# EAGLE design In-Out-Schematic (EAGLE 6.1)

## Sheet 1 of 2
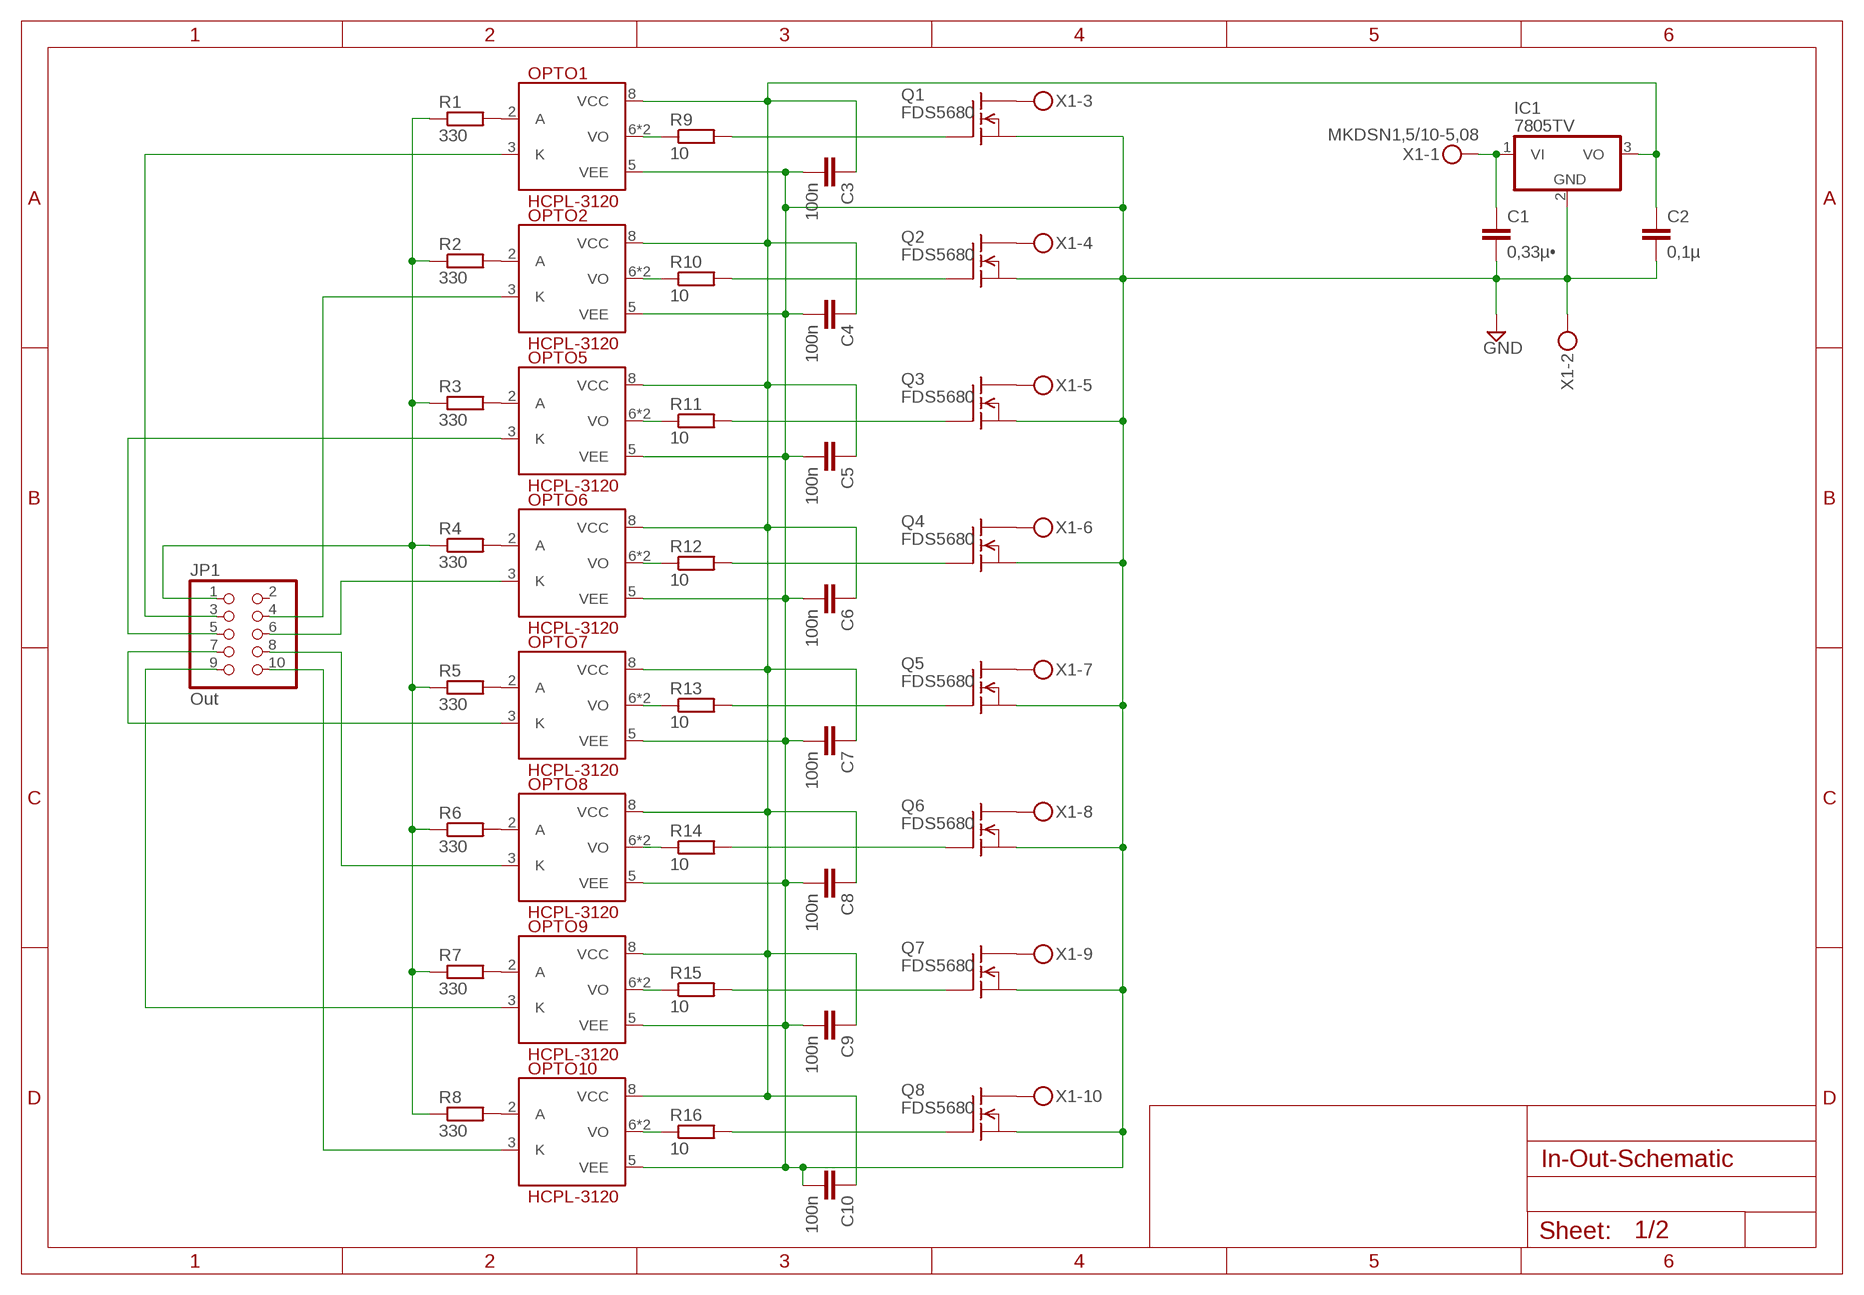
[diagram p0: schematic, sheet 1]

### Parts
C1  0,33µ•  C-EUC0805  [C0805]
C2  0,1µ  C-EUC0402  [C0402]
C3  100n  C-EUC0402  [C0402]
C4  100n  C-EUC0402  [C0402]
C5  100n  C-EUC0402  [C0402]
C6  100n  C-EUC0402  [C0402]
C7  100n  C-EUC0402  [C0402]
C8  100n  C-EUC0402  [C0402]
C9  100n  C-EUC0402  [C0402]
C10  100n  C-EUC0402  [C0402]
IC1  7805TV  [TO220V]
JP1  Out  PINHD-2X5  [2X05]
OPTO1  HCPL-3120  [HCPL-3120-SOIC-8]
OPTO2  HCPL-3120  [HCPL-3120-SOIC-8]
OPTO5  HCPL-3120  [HCPL-3120-SOIC-8]
OPTO6  HCPL-3120  [HCPL-3120-SOIC-8]
OPTO7  HCPL-3120  [HCPL-3120-SOIC-8]
OPTO8  HCPL-3120  [HCPL-3120-SOIC-8]
OPTO9  HCPL-3120  [HCPL-3120-SOIC-8]
OPTO10  HCPL-3120  [HCPL-3120-SOIC-8]
Q1  FDS5680  [SO-8]
Q2  FDS5680  [SO-8]
Q3  FDS5680  [SO-8]
Q4  FDS5680  [SO-8]
Q5  FDS5680  [SO-8]
Q6  FDS5680  [SO-8]
Q7  FDS5680  [SO-8]
Q8  FDS5680  [SO-8]
R1  330  R-EU_R0603  [R0603]
R2  330  R-EU_R0603  [R0603]
R3  330  R-EU_R0603  [R0603]
R4  330  R-EU_R0603  [R0603]
R5  330  R-EU_R0603  [R0603]
R6  330  R-EU_R0603  [R0603]
R7  330  R-EU_R0603  [R0603]
R8  330  R-EU_R0603  [R0603]
R9  10  R-EU_R1206  [R1206]
R10  10  R-EU_R1206  [R1206]
R11  10  R-EU_R1206  [R1206]
R12  10  R-EU_R1206  [R1206]
R13  10  R-EU_R1206  [R1206]
R14  10  R-EU_R1206  [R1206]
R15  10  R-EU_R1206  [R1206]
R16  10  R-EU_R1206  [R1206]
X1  MKDSN1,5/10-5,08  [MKDSN1,5/10-5,08]

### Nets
GND: C1.2 C2.2 C3.2 C4.2 C5.2 C6.2 C7.2 C8.2 C9.2 C10.2 IC1.2(GND) OPTO1.5(VEE) OPTO2.5(VEE) OPTO5.5(VEE) OPTO6.5(VEE) OPTO7.5(VEE) OPTO8.5(VEE) OPTO9.5(VEE) OPTO10.5(VEE) Q1.1(S) Q1.2(S) Q1.3(S) Q2.1(S) Q2.2(S) Q2.3(S) Q3.1(S) Q3.2(S) Q3.3(S) Q4.1(S) Q4.2(S) Q4.3(S) Q5.1(S) Q5.2(S) Q5.3(S) Q6.1(S) Q6.2(S) Q6.3(S) Q7.1(S) Q7.2(S) Q7.3(S) Q8.1(S) Q8.2(S) Q8.3(S) X1.2
N$2 [Power]: C1.1 IC1.1(VI) X1.1
N$3: Q1.5(D) Q1.6(D) Q1.7(D) Q1.8(D) X1.3
N$4: Q2.5(D) Q2.6(D) Q2.7(D) Q2.8(D) X1.4
N$5: Q3.5(D) Q3.6(D) Q3.7(D) Q3.8(D) X1.5
N$6: Q4.5(D) Q4.6(D) Q4.7(D) Q4.8(D) X1.6
N$7: Q5.5(D) Q5.6(D) Q5.7(D) Q5.8(D) X1.7
N$8: Q6.5(D) Q6.6(D) Q6.7(D) Q6.8(D) X1.8
N$9: Q7.5(D) Q7.6(D) Q7.7(D) Q7.8(D) X1.9
N$10: Q8.5(D) Q8.6(D) Q8.7(D) Q8.8(D) X1.10
N$11: OPTO1.2(A) R1.2
N$12: OPTO2.2(A) R2.2
N$13: OPTO5.2(A) R3.2
N$14: OPTO6.2(A) R4.2
N$15: OPTO7.2(A) R5.2
N$16: OPTO8.2(A) R6.2
N$17: OPTO9.2(A) R7.2
N$18: OPTO10.2(A) R8.2
N$19: JP1.1 R1.1 R2.1 R3.1 R4.1 R5.1 R6.1 R7.1 R8.1
N$20: JP1.5 OPTO5.3(K)
N$21: JP1.3 OPTO1.3(K)
N$22: JP1.4 OPTO2.3(K)
N$23: JP1.6 OPTO6.3(K)
N$24: JP1.7 OPTO7.3(K)
N$25: JP1.8 OPTO8.3(K)
N$26: JP1.9 OPTO9.3(K)
N$27: JP1.10 OPTO10.3(K)
N$28: OPTO1.6(VO) OPTO1.7(VO) R9.1
N$29: Q1.4(G) R9.2
N$30: OPTO2.6(VO) OPTO2.7(VO) R10.1
N$31: Q2.4(G) R10.2
N$32: OPTO5.6(VO) OPTO5.7(VO) R11.1
N$33: Q3.4(G) R11.2
N$34: OPTO6.6(VO) OPTO6.7(VO) R12.1
N$35: Q4.4(G) R12.2
N$36: OPTO7.6(VO) OPTO7.7(VO) R13.1
N$37: Q5.4(G) R13.2
N$38: Q6.4(G) R14.2
N$39: OPTO8.6(VO) OPTO8.7(VO) R14.1
N$40: OPTO9.6(VO) OPTO9.7(VO) R15.1
N$41: Q7.4(G) R15.2
N$42: OPTO10.6(VO) OPTO10.7(VO) R16.1
N$59: Q8.4(G) R16.2
N$71 [Power]: C2.1 C3.1 C4.1 C5.1 C6.1 C7.1 C8.1 C9.1 C10.1 IC1.3(VO) OPTO1.8(VCC) OPTO2.8(VCC) OPTO5.8(VCC) OPTO6.8(VCC) OPTO7.8(VCC) OPTO8.8(VCC) OPTO9.8(VCC) OPTO10.8(VCC)
Unconnected: JP1.2

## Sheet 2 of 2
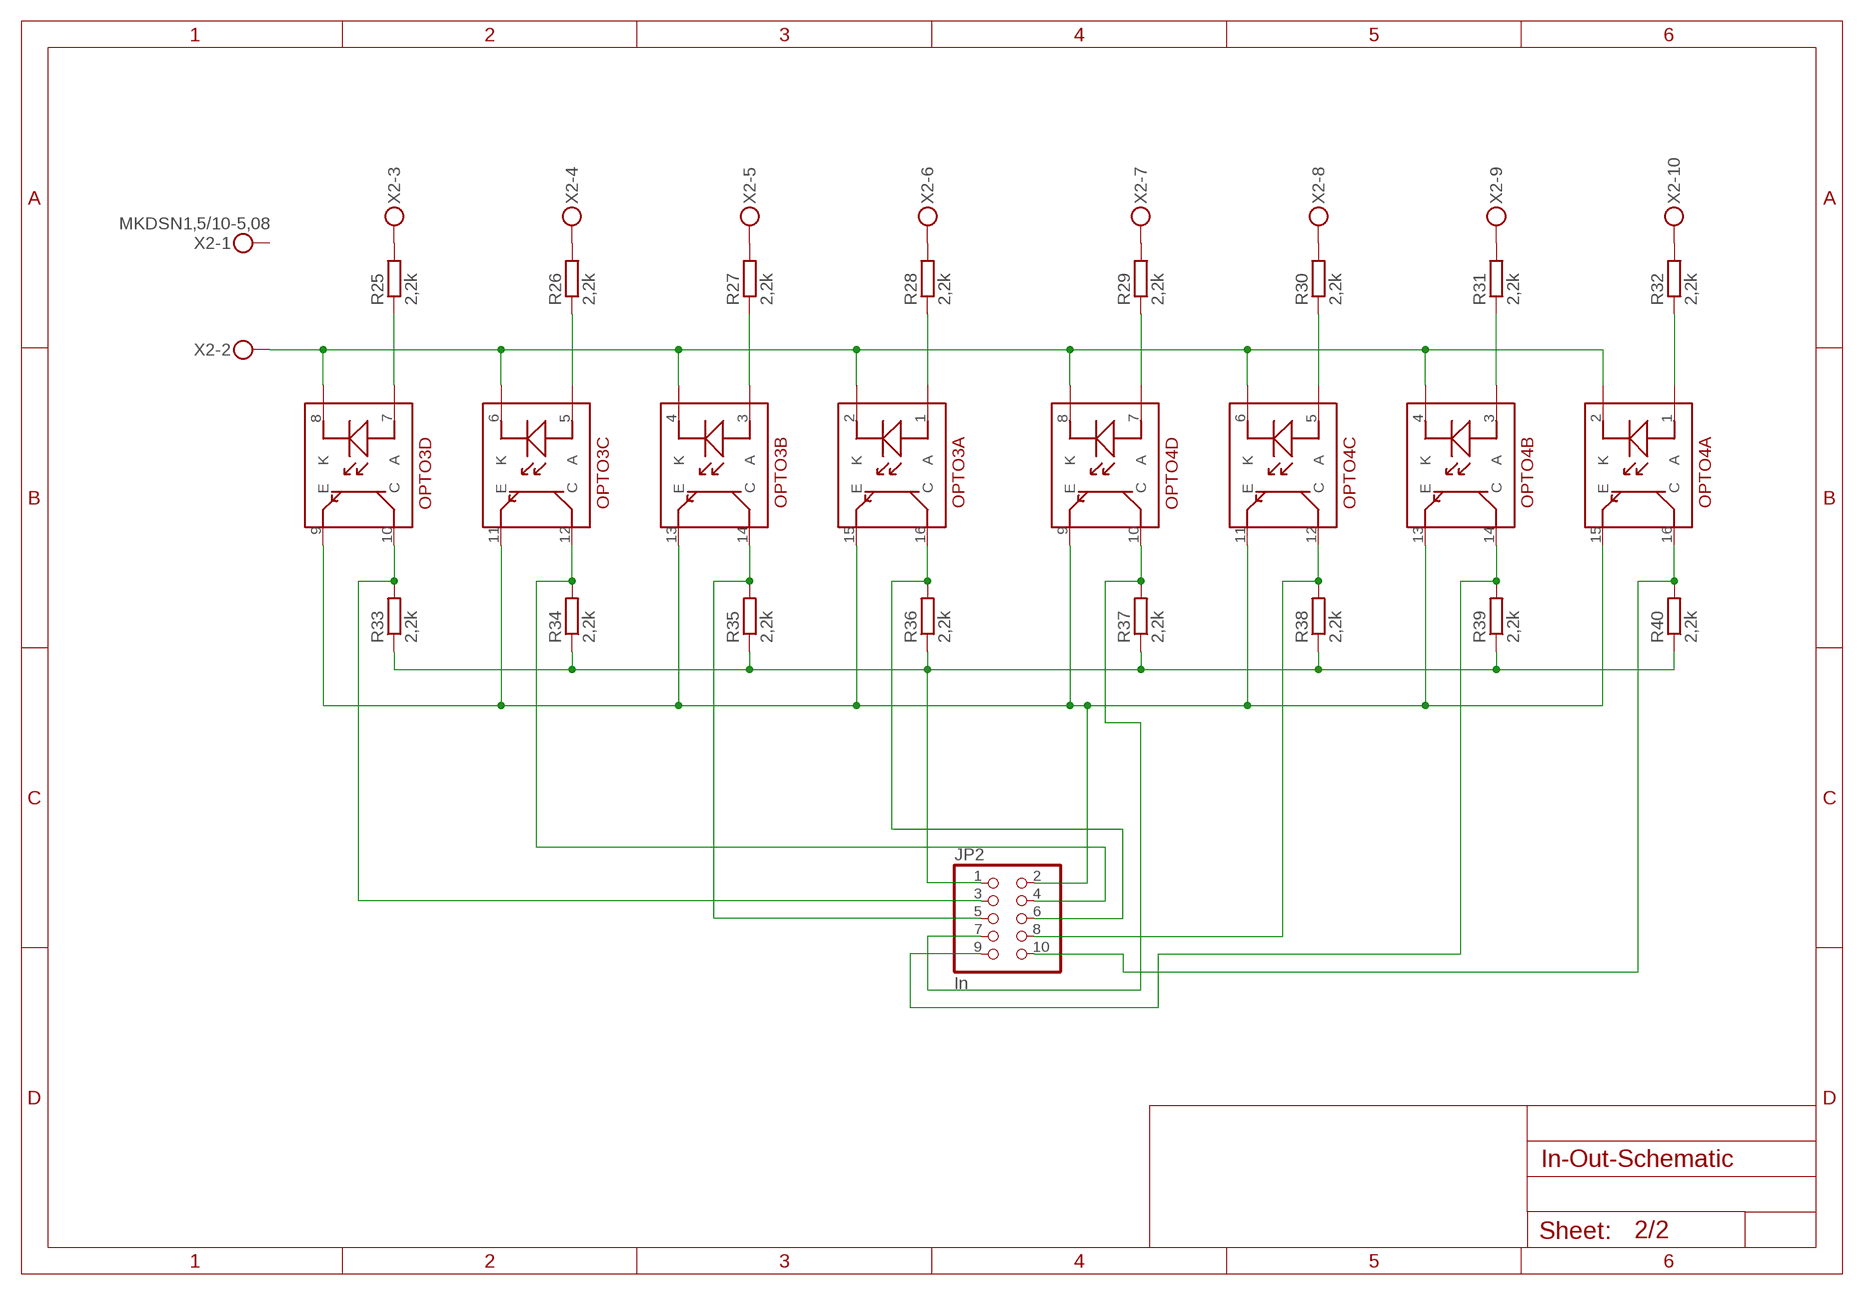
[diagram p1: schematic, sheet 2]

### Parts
JP2  In  PINHD-2X5  [2X05]
OPTO3  QUAD-OPTO_ACPL-247  [SOIC-16]
OPTO4  QUAD-OPTO_ACPL-247  [SOIC-16]
R25  2,2k  R-EU_R0805  [R0805]
R26  2,2k  R-EU_R0805  [R0805]
R27  2,2k  R-EU_R0805  [R0805]
R28  2,2k  R-EU_R0805  [R0805]
R29  2,2k  R-EU_R0805  [R0805]
R30  2,2k  R-EU_R0805  [R0805]
R31  2,2k  R-EU_R0805  [R0805]
R32  2,2k  R-EU_R0805  [R0805]
R33  2,2k  R-EU_R0805  [R0805]
R34  2,2k  R-EU_R0805  [R0805]
R35  2,2k  R-EU_R0805  [R0805]
R36  2,2k  R-EU_R0805  [R0805]
R37  2,2k  R-EU_R0805  [R0805]
R38  2,2k  R-EU_R0805  [R0805]
R39  2,2k  R-EU_R0805  [R0805]
R40  2,2k  R-EU_R0805  [R0805]
X2  MKDSN1,5/10-5,08  [MKDSN1,5/10-5,08]

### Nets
N$43: OPTO3.7(D:A) R25.1
N$44: OPTO3.1(A:A) R28.1
N$45: OPTO3.5(C:A) R26.1
N$46: OPTO3.3(B:A) R27.1
N$47: OPTO3.2(A:K) OPTO3.4(B:K) OPTO3.6(C:K) OPTO3.8(D:K) OPTO4.2(A:K) OPTO4.4(B:K) OPTO4.6(C:K) OPTO4.8(D:K) X2.2
N$48: OPTO4.7(D:A) R29.1
N$49: OPTO4.5(C:A) R30.1
N$50: OPTO4.3(B:A) R31.1
N$51: OPTO4.1(A:A) R32.1
N$52: JP2.3 OPTO3.10(D:C) R33.2
N$53: JP2.4 OPTO3.12(C:C) R34.2
N$54: JP2.5 OPTO3.14(B:C) R35.2
N$55: JP2.6 OPTO3.16(A:C) R36.2
N$56: JP2.7 OPTO4.10(D:C) R37.2
N$57: JP2.8 OPTO4.12(C:C) R38.2
N$58: JP2.10 OPTO4.16(A:C) R40.2
N$60: R25.2 X2.3
N$61: R26.2 X2.4
N$62: R27.2 X2.5
N$63: R28.2 X2.6
N$64: R29.2 X2.7
N$65: R30.2 X2.8
N$66: R31.2 X2.9
N$67: R32.2 X2.10
N$68: JP2.1 R33.1 R34.1 R35.1 R36.1 R37.1 R38.1 R39.1 R40.1
N$69: JP2.2 OPTO3.9(D:E) OPTO3.11(C:E) OPTO3.13(B:E) OPTO3.15(A:E) OPTO4.9(D:E) OPTO4.11(C:E) OPTO4.13(B:E) OPTO4.15(A:E)
N$77: JP2.9 OPTO4.14(B:C) R39.2
Unconnected: X2.1

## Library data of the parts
C1-C10 = rcl:C-EU: CAPACITOR, European symbol
IC1 = linear:78*: Positive VOLTAGE REGULATOR Source: http://cache.national.com/ds/LM/LM78L05.pdf http://www.fairchildsemi.com/ds/LM/LM7805.pdf
JP1 JP2 = pinhead:PINHD-2X5: PIN HEADER
OPTO1 OPTO2 OPTO5-OPTO10 = Bachelorarbeit_lib_Jonas:HCPL-3120: HCPL-3120 Gate Driver Opto
OPTO3 OPTO4 = Bachelorarbeit_lib_Jonas:QUAD-OPTO_ACPL-247: 4-fach Optokoppler AVAGO ACPL-247 SOIC-16 Package
Q1-Q8 = transistor-fet:FDS5680: 60V N-Channel PowerTrench TM MOSFET FAIRCHILD FDS5680.pdf
R1-R16 R25-R40 = rcl:R-EU_: RESISTOR, European symbol
X1 X2 = con-phoenix-508:MKDSN1,5/10-5,08: MKDSN 1,5/10-5,08 Printklemme Nennstrom: 13,5 A Nennspannung: 250 V Rastermaß: 5,08 mm Polzahl: 10 Anschlussart: Schraubanschluss Montage: Löten Anschlussrichtung Leiter/Platine: 0 ° Artikelnummer: 1729209 Source: http://eshop.phoenixcontact.com .. 1729209.pdf; MPN: SMKDSN1,5/10-5,08; OC_FARNELL: 1792913; OC_NEWARK: 70R0297

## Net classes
1 Power: width 0.508 mm, clearance 0.305 mm

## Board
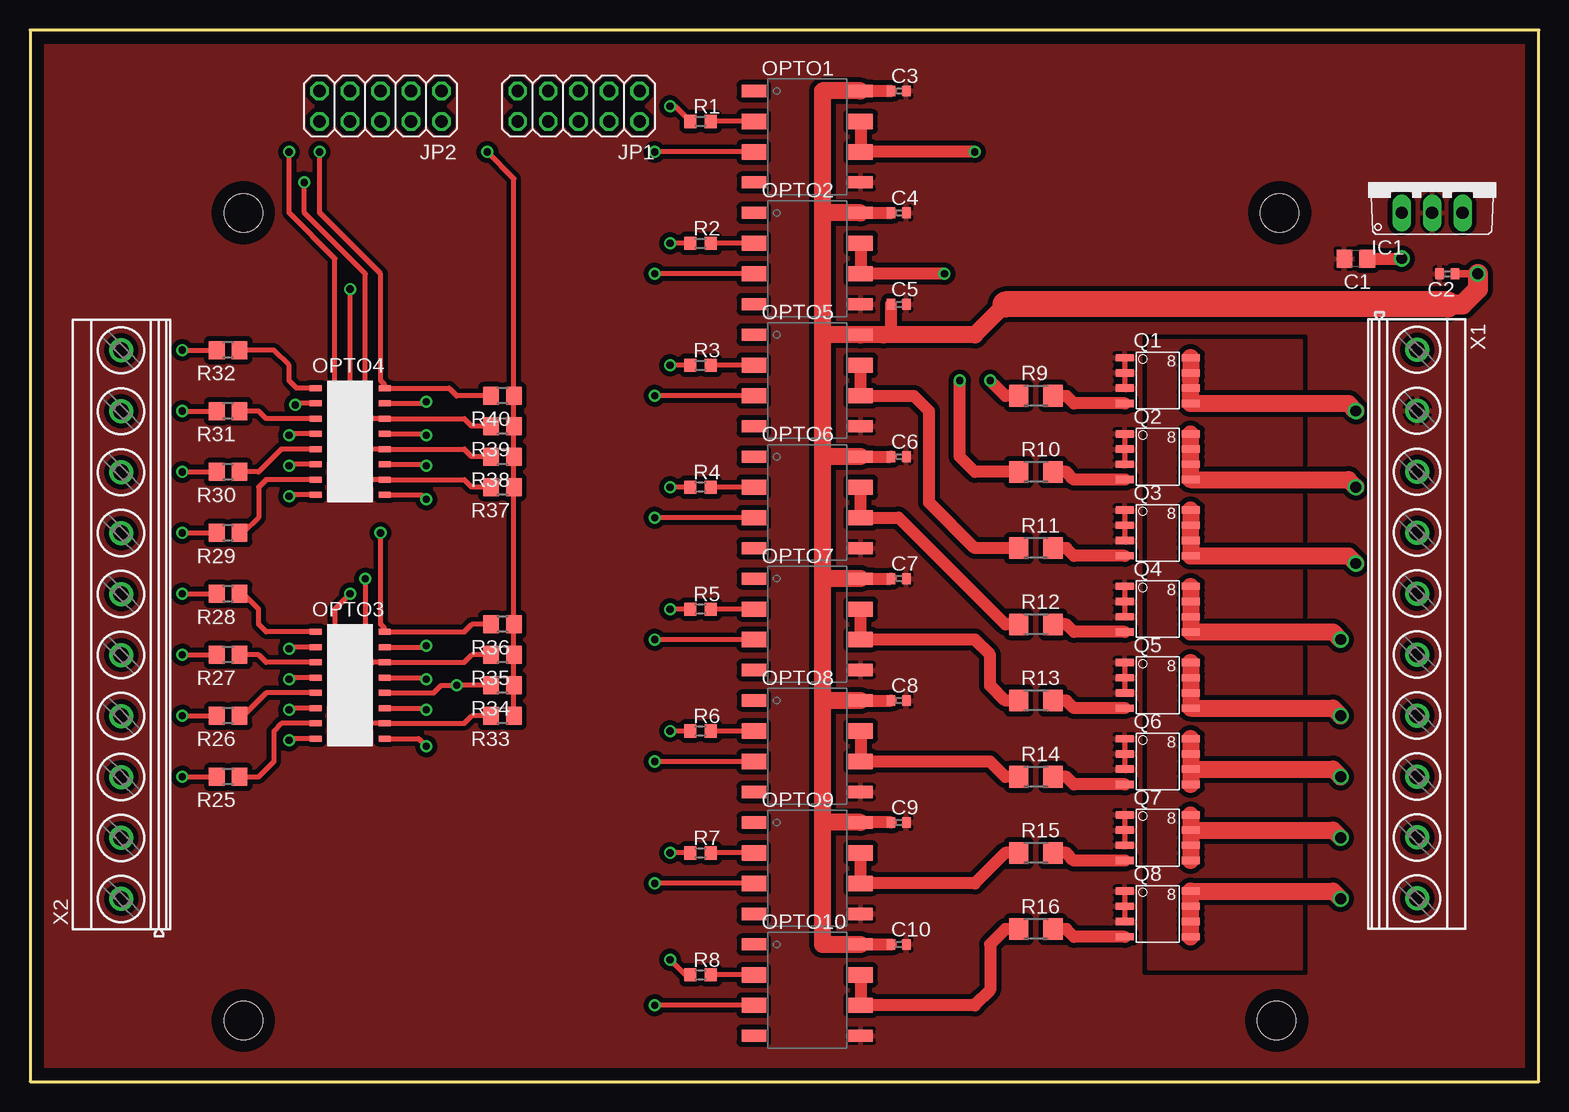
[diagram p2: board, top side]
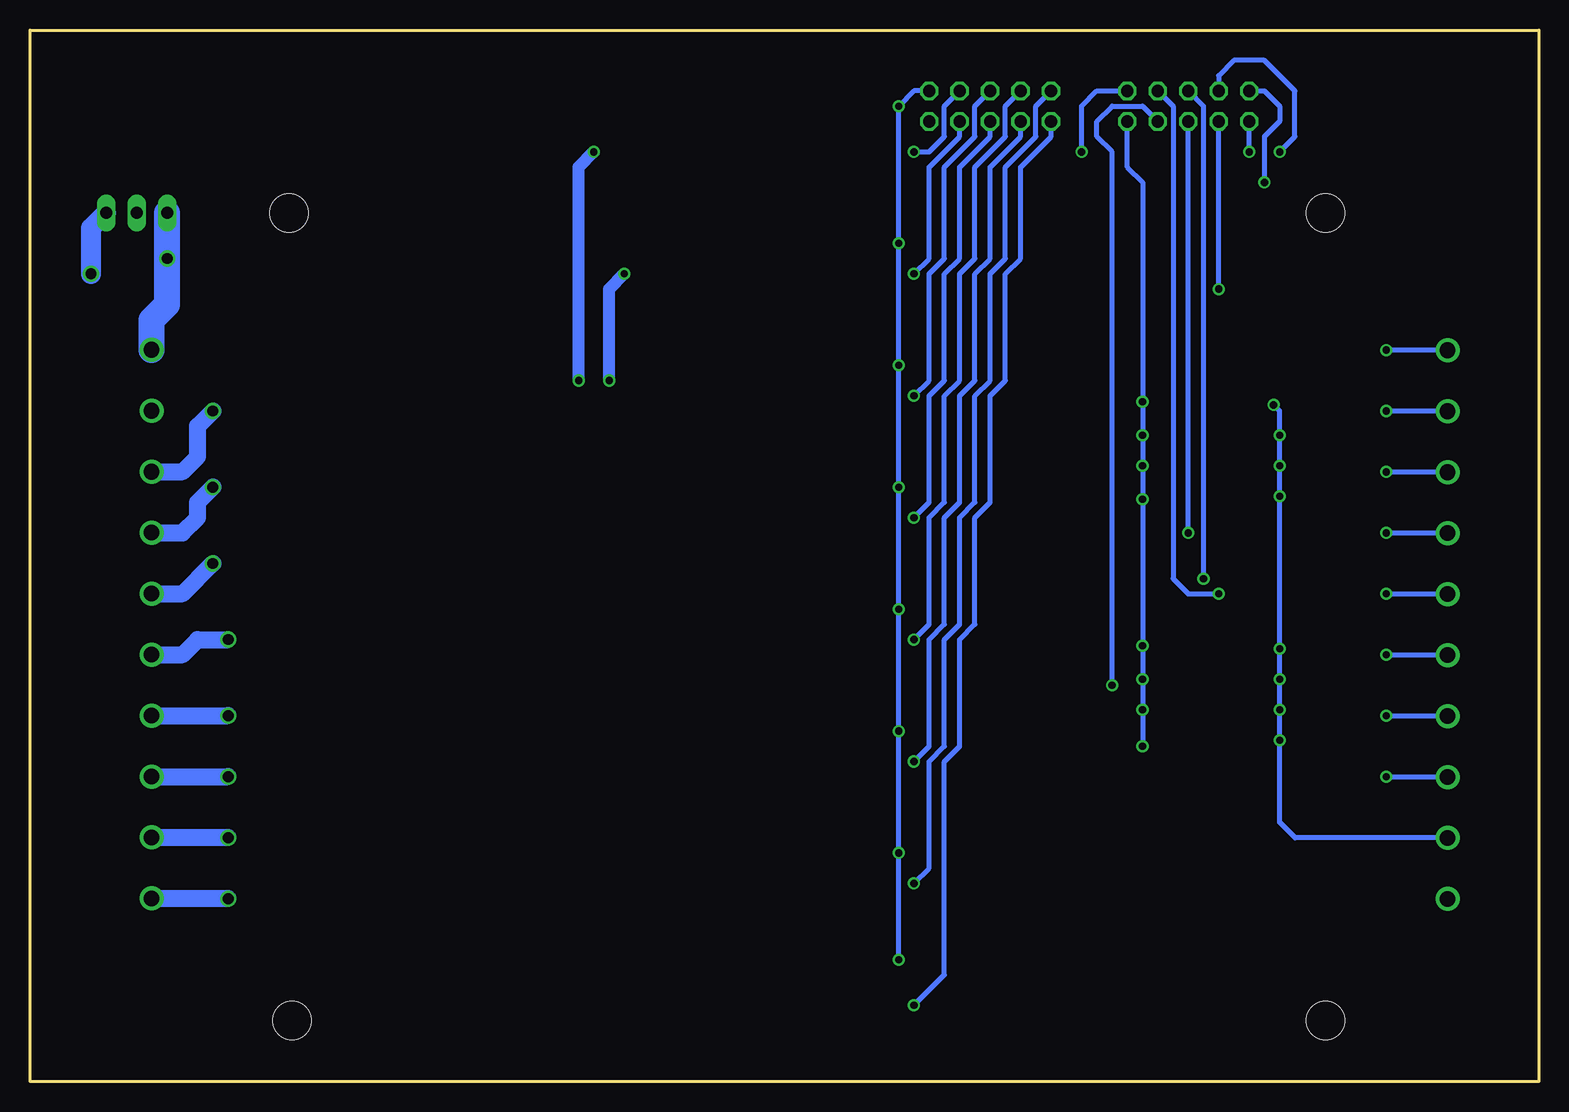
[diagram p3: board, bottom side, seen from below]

Size 125.73 x 87.63 mm. Coordinates in mm from the lower left corner, seen from the top.
Outline: 0,0 125.73,0 125.73,87.63 0,87.63 0,0
Copper layers (1*16): Top 0.035mm / dielectric 1.5mm / Bottom 0.035mm
Design rules: minimum track width 10mil, minimum drill 23mil, track to track 16mil, track to pad 12mil, pad to pad 16mil, via to via 16mil, smd to smd 8mil, copper to edge 40mil, drill to drill 8mil, minimum pad ring 10mil, minimum via ring 8mil, stop-mask expansion 4mil, vias tented up to drill 0mil, thermal gap 10mil
Holes 3.2 mm at 17.78,5.08 17.78,72.39 103.89,5.08 104.14,72.39

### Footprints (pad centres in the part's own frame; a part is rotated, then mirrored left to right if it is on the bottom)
C0805 = smd 1.3 x 1.5: 1 -0.95,0; 2 0.95,0
C0402 = smd 0.7 x 0.9: 1 -0.65,0; 2 0.65,0
TO220V = drill 1.016 long: 1 -2.54,-2.54; 2 0,-2.54; 3 2.54,-2.54
2X05 = drill 1.016 octagon: 1 -5.08,-1.27; 2 -5.08,1.27; 3 -2.54,-1.27; 4 -2.54,1.27; 5 0,-1.27; 6 0,1.27; 7 2.54,-1.27; 8 2.54,1.27; 9 5.08,-1.27; 10 5.08,1.27
HCPL-3120-SOIC-8 = smd 1.016 x 2.032: 1 -3.81,-4.445; 4 3.81,-4.445; 5 3.81,4.445; 8 -3.81,4.445 | smd 1.27 x 2.032: 2 -1.27,-4.445; 3 1.27,-4.445; 6 1.27,4.445; 7 -1.27,4.445
SOIC-16 = smd 0.5 x 1: 1 -4.445,-2.875; 2 -3.175,-2.875; 3 -1.905,-2.875; 4 -0.635,-2.875; 5 0.635,-2.875; 6 1.905,-2.875; 7 3.175,-2.875; 8 4.445,-2.875; 9 4.445,2.875; 10 3.175,2.875; 11 1.905,2.875; 12 0.635,2.875; 13 -0.635,2.875; 14 -1.905,2.875; 15 -3.175,2.875; 16 -4.445,2.875
SO-8 = smd 1.524 x 0.61: 1 -2.743,1.905; 2 -2.743,0.635; 3 -2.743,-0.635; 4 -2.743,-1.905; 5 2.743,-1.905; 6 2.743,-0.635; 7 2.743,0.635; 8 2.743,1.905
R0603 = smd 1 x 1.1: 1 -0.85,0; 2 0.85,0
R1206 = smd 1.6 x 1.803: 1 -1.422,0; 2 1.422,0
R0805 = smd 1.3 x 1.5: 1 -0.95,0; 2 0.95,0
MKDSN1,5/10-5,08 = drill 1.3 pad 2: 1 -22.881,0.025; 2 -17.801,0.025; 3 -12.721,0.025; 4 -7.641,0.025; 5 -2.561,0.025; 6 2.519,0.025; 7 7.599,0.025; 8 12.679,0.025; 9 17.759,0.025; 10 22.839,0.025

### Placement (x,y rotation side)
C1  110.49,68.58 180 top
C2  118.11,67.31 180 top
C3  72.39,82.55 0 top
C4  72.39,72.39 0 top
C5  72.39,64.77 0 top
C6  72.39,52.07 0 top
C7  72.39,41.91 0 top
C8  72.39,31.75 0 top
C9  72.39,21.59 0 top
C10  72.39,11.43 0 top
IC1  116.84,74.93 0 top
JP1  45.72,81.28 180 top
JP2  29.21,81.28 180 top
OPTO1  64.77,78.74 270 top
OPTO2  64.77,68.58 270 top
OPTO3  26.67,33.02 270 top
OPTO4  26.67,53.34 270 top
OPTO5  64.77,58.42 270 top
OPTO6  64.77,48.26 270 top
OPTO7  64.77,38.1 270 top
OPTO8  64.77,27.94 270 top
OPTO9  64.77,17.78 270 top
OPTO10  64.77,7.62 270 top
Q1  93.98,58.42 0 top
Q2  93.98,52.07 0 top
Q3  93.98,45.72 0 top
Q4  93.98,39.37 0 top
Q5  93.98,33.02 0 top
Q6  93.98,26.67 0 top
Q7  93.98,20.32 0 top
Q8  93.98,13.97 0 top
R1  55.88,80.01 0 top
R2  55.88,69.85 0 top
R3  55.88,59.69 0 top
R4  55.88,49.53 0 top
R5  55.88,39.37 0 top
R6  55.88,29.21 0 top
R7  55.88,19.05 0 top
R8  55.88,8.89 0 top
R9  83.82,57.15 0 top
R10  83.82,50.8 0 top
R11  83.82,44.45 0 top
R12  83.82,38.1 0 top
R13  83.82,31.75 0 top
R14  83.82,25.4 0 top
R15  83.82,19.05 0 top
R16  83.82,12.7 0 top
R25  16.51,25.4 180 top
R26  16.51,30.48 180 top
R27  16.51,35.56 180 top
R28  16.51,40.64 180 top
R29  16.51,45.72 180 top
R30  16.51,50.8 180 top
R31  16.51,55.88 180 top
R32  16.51,60.96 180 top
R33  39.37,30.48 180 top
R34  39.37,33.02 180 top
R35  39.37,35.56 180 top
R36  39.37,38.1 180 top
R37  39.37,49.53 180 top
R38  39.37,52.07 180 top
R39  39.37,54.61 180 top
R40  39.37,57.15 180 top
X1  115.57,38.1 270 top
X2  7.62,38.1 90 top

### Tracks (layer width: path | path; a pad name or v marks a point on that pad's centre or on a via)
COOLAREA
  pour Top (rank 2, no thermals): 93.47,61.72 105.92,61.72 105.92,53.85 105.92,41.15 105.92,28.7 105.92,17.27 105.92,9.4 93.47,9.4 93.22,9.4 93.22,16.76 93.22,25.91 93.22,38.86 93.22,51.56 93.22,61.72
GND
  Top 0.406: Q1.1 Q1.2 Q1.3 | Q2.1 Q2.2 Q2.3 | Q3.1 Q3.2 Q3.3 | Q4.1 Q4.2 Q4.3 | Q5.1 Q5.2 Q5.3 | Q6.1 Q6.2 Q6.3 | Q7.1 Q7.2 Q7.3 | Q8.1 Q8.2 Q8.3
  pour Top (rank 6): 1.27,1.27 124.46,1.27 124.46,86.36 1.27,86.36
N$2  (via drill 0.9)
  Top 1.016: C1.1 v114.3,68.58
  Bottom 2.184: X1.1 115.59,63.48 114.3,64.77 v114.3,68.58 IC1.1
N$3  (via drill 0.9)
  Top 0.406: Q1.6 96.72,58.42
  Top 1.422: v110.49,55.88 109.85,56.52 Q1.5 Q1.6 | 96.72,58.42 Q1.7 Q1.8
  Bottom 1.422: X1.3 113.01,50.82 111.76,52.07 111.76,54.61 v110.49,55.88
N$4  (via drill 0.9)
  Top 1.422: v110.49,49.53 109.85,50.17 Q2.5 Q2.6 Q2.7 Q2.8
  Bottom 0.406: 113.05,45.74 113.03,45.72
  Bottom 1.422: X1.4 113.05,45.74 | 113.03,45.72 111.76,46.99 111.76,48.26 v110.49,49.53
N$5  (via drill 0.9)
  Top 1.422: Q3.8 Q3.7 Q3.6 Q3.5 109.85,43.82 v110.49,43.18
  Bottom 1.422: X1.5 113.01,40.66 v110.49,43.18
N$6  (via drill 0.9)
  Top 1.422: Q4.8 Q4.7 Q4.6 Q4.5 108.58,37.47 v109.22,36.83
  Bottom 1.422: X1.6 113.01,35.58 111.76,36.83 v109.22,36.83
N$7  (via drill 0.9)
  Top 1.422: Q5.8 Q5.7 Q5.6 Q5.5 108.58,31.11 v109.22,30.48
  Bottom 0.406: 109.24,30.5 v109.22,30.48
  Bottom 1.422: X1.7 109.24,30.5
N$8  (via drill 0.9)
  Top 1.422: Q6.8 Q6.7 Q6.6 | Q6.6 Q6.5 | Q6.6 108.58,26.04 v109.22,25.4
  Bottom 0.406: 109.24,25.42 v109.22,25.4
  Bottom 1.422: X1.8 109.24,25.42
N$9  (via drill 0.9)
  Top 1.422: Q7.8 Q7.7 | Q7.7 Q7.6 Q7.5 | Q7.7 108.58,20.95 v109.22,20.32
  Bottom 0.406: 109.24,20.34 v109.22,20.32
  Bottom 1.422: X1.9 109.24,20.34
N$10  (via drill 0.9)
  Top 1.422: Q8.5 Q8.6 Q8.7 Q8.8 108.58,15.88 v109.22,15.24
  Bottom 0.406: 109.24,15.26 v109.22,15.24
  Bottom 1.422: X1.10 109.24,15.26
N$11
  Top 0.406: OPTO1.2 R1.2
N$12
  Top 0.406: OPTO2.2 R2.2
N$13
  Top 0.406: OPTO5.2 R3.2
N$14
  Top 0.406: OPTO6.2 R4.2
N$15
  Top 0.406: OPTO7.2 R5.2
N$16
  Top 0.406: OPTO8.2 R6.2
N$17
  Top 0.406: OPTO9.2 R7.2
N$18
  Top 0.406: OPTO10.2 R8.2
N$19  (via drill 0.6)
  Top 0.406: v53.34,81.28 53.76,81.28 R1.1 | R8.1 54.61,8.89 v53.34,10.16 | R2.1 v53.34,69.85 | R3.1 v53.34,59.69 | R4.1 v53.34,49.53 | R5.1 v53.34,39.37 | R6.1 v53.34,29.21 | R7.1 v53.34,19.05
  Bottom 0.406: JP1.1 52.07,82.55 v53.34,81.28 v53.34,69.85 v53.34,59.69 v53.34,49.53 v53.34,39.37 v53.34,29.21 v53.34,19.05 v53.34,10.16
N$20  (via drill 0.6)
  Top 0.406: OPTO5.3 v52.07,57.15
  Bottom 0.406: v52.07,57.15 50.8,58.42 50.8,67.31 49.53,68.58 49.53,76.2 46.99,78.74 46.99,81.28 JP1.5
N$21  (via drill 0.6)
  Top 0.406: OPTO1.3 v52.07,77.47
  Bottom 0.406: v52.07,77.47 50.8,77.47 49.53,78.74 49.53,81.28 JP1.3
N$22  (via drill 0.6)
  Top 0.406: OPTO2.3 v52.07,67.31
  Bottom 0.406: v52.07,67.31 50.8,68.58 50.8,76.2 48.26,78.74 JP1.4
N$23  (via drill 0.6)
  Top 0.406: OPTO6.3 v52.07,46.99
  Bottom 0.406: v52.07,46.99 50.8,48.26 50.8,57.15 49.53,58.42 49.53,67.31 48.26,68.58 48.26,76.2 45.72,78.74 JP1.6
N$24  (via drill 0.6)
  Top 0.406: OPTO7.3 v52.07,36.83
  Bottom 0.406: v52.07,36.83 50.8,38.1 50.8,46.99 49.53,48.26 49.53,57.15 48.26,58.42 48.26,67.31 46.99,68.58 46.99,76.2 44.45,78.74 44.45,81.28 JP1.7
N$25  (via drill 0.6)
  Top 0.406: OPTO8.3 v52.07,26.67
  Bottom 0.406: v52.07,26.67 50.8,27.94 50.8,36.83 49.53,38.1 49.53,46.99 48.26,48.26 48.26,57.15 46.99,58.42 46.99,67.31 45.72,68.58 45.72,76.2 43.18,78.74 JP1.8
N$26  (via drill 0.6)
  Top 0.406: OPTO9.3 v52.07,16.51
  Bottom 0.406: v52.07,16.51 50.8,17.78 50.8,26.67 49.53,27.94 49.53,36.83 48.26,38.1 48.26,46.99 46.99,48.26 46.99,57.15 45.72,58.42 45.72,67.31 44.45,68.58 44.45,76.2 41.91,78.74 41.91,81.28 JP1.9
N$27  (via drill 0.6)
  Top 0.406: OPTO10.3 v52.07,6.35
  Bottom 0.406: v52.07,6.35 49.53,8.89 49.53,26.67 48.26,27.94 48.26,36.83 46.99,38.1 46.99,46.99 45.72,48.26 45.72,57.15 44.45,58.42 44.45,67.31 43.18,68.58 43.18,76.2 40.64,78.74 JP1.10
N$28  (via drill 0.6)
  Top 1.016: R9.1 81.28,57.15 v80.01,58.42 | v78.74,77.47 OPTO1.6 OPTO1.7
  Bottom 1.016: v80.01,58.42 80.01,76.2 v78.74,77.47
N$29
  Top 1.016: R9.2 86.36,57.15 86.99,56.52 Q1.4
N$30  (via drill 0.6)
  Top 1.016: R10.1 78.74,50.8 77.47,52.07 v77.47,58.42 | v76.2,67.31 OPTO2.6 OPTO2.7
  Bottom 1.016: v77.47,58.42 77.47,66.04 v76.2,67.31
N$31
  Top 1.016: Q2.4 86.99,50.17 86.36,50.8 R10.2
N$32
  Top 1.016: R11.1 78.74,44.45 74.93,48.26 74.93,55.88 73.66,57.15 OPTO5.6 OPTO5.7
N$33
  Top 1.016: Q3.4 86.99,43.82 86.36,44.45 R11.2
N$34
  Top 1.016: OPTO6.7 OPTO6.6 72.39,46.99 81.28,38.1 R12.1
N$35
  Top 1.016: Q4.4 86.99,37.47 86.36,38.1 R12.2
N$36
  Top 1.016: R13.1 81.28,31.75 80.01,33.02 80.01,35.56 78.74,36.83 OPTO7.6 OPTO7.7
N$37
  Top 1.016: Q5.4 86.99,31.11 86.36,31.75 R13.2
N$38
  Top 1.016: Q6.4 86.99,24.77 86.36,25.4 R14.2
N$39
  Top 1.016: R14.1 81.28,25.4 80.01,26.67 OPTO8.6 OPTO8.7
N$40
  Top 1.016: R15.1 81.28,19.05 78.74,16.51 OPTO9.6 OPTO9.7
N$41
  Top 1.016: Q7.4 86.99,18.41 86.36,19.05 R15.2
N$42
  Top 1.016: R16.1 81.28,12.7 80.01,11.43 80.01,7.62 78.74,6.35 OPTO10.6 OPTO10.7
N$43
  Top 0.406: R25.1 19.05,25.4 20.32,26.67 20.32,29.21 20.95,29.84 OPTO3.7
N$44
  Top 0.406: OPTO3.1 19.68,37.47 19.05,38.1 19.05,39.37 17.78,40.64 R28.1
N$45
  Top 0.406: R26.1 17.78,30.48 19.68,32.38 OPTO3.5
N$46
  Top 0.406: OPTO3.3 19.68,34.93 19.05,35.56 R27.1
N$47  (via drill 0.6)
  Top 0.406: OPTO4.2 22.22,56.52 v22.1,56.39 | OPTO4.4 21.72,53.98 v21.59,53.85 | OPTO4.6 21.72,51.44 v21.59,51.31 | OPTO4.8 21.72,48.9 v21.59,48.77 | OPTO3.2 21.72,36.2 v21.59,36.07 | OPTO3.4 21.72,33.66 v21.59,33.53 | OPTO3.6 21.72,31.11 v21.59,30.99 | OPTO3.8 21.72,28.57 v21.59,28.45
  Bottom 0.406: X2.2 20.3,20.3 21.59,21.59 v21.59,28.45 v21.59,30.99 v21.59,33.53 v21.59,36.07 v21.59,48.77 v21.59,51.31 v21.59,53.85 21.59,55.88 v22.1,56.39
N$48
  Top 0.406: OPTO4.7 19.68,50.17 19.05,49.53 19.05,46.99 17.78,45.72 R29.1
N$49
  Top 0.406: OPTO4.5 20.95,52.71 19.05,50.8 R30.1
N$50
  Top 0.406: OPTO4.3 19.68,55.25 19.05,55.88 R31.1
N$51
  Top 0.406: OPTO4.1 22.22,57.79 21.59,58.42 21.59,59.69 20.32,60.96 R32.1
N$52  (via drill 0.6)
  Top 0.406: R33.2 36.83,30.48 36.2,29.84 OPTO3.10 27.3,29.84 25.4,31.75 25.4,39.37 v26.67,40.64
  Bottom 0.406: JP2.3 30.48,81.28 30.48,41.91 29.21,40.64 v26.67,40.64
N$53  (via drill 0.6)
  Top 0.406: OPTO3.12 33.66,32.38 34.29,33.02 v35.56,33.02 R34.2
  Bottom 0.406: v35.56,33.02 35.56,77.47 36.83,78.74 36.83,80.01 35.56,81.28 33.02,81.28 JP2.4
N$54  (via drill 0.6)
  Top 0.406: R35.2 36.83,35.56 36.2,34.93 OPTO3.14 28.57,34.93 27.94,35.56 v27.94,41.91
  Bottom 0.406: JP2.5 27.94,81.28 v27.94,41.91
N$55  (via drill 0.6)
  Top 0.406: R36.2 36.83,38.1 36.2,37.47 OPTO3.16 29.54,37.77 29.21,38.1 v29.21,45.72
  Bottom 0.406: v29.21,45.72 JP2.6
N$56  (via drill 0.6)
  Top 0.406: R37.2 36.83,49.53 36.2,50.17 OPTO4.10 27.3,50.17 25.4,52.07 25.4,68.58 21.59,72.39 v21.59,77.47
  Bottom 0.406: JP2.7 26.67,83.82 25.4,85.09 22.86,85.09 20.32,82.55 20.32,78.74 v21.59,77.47
N$57  (via drill 0.6)
  Top 0.406: R38.2 36.83,52.07 36.2,52.71 OPTO4.12 27.3,52.71 26.67,53.34 v26.67,66.04
  Bottom 0.406: v26.67,66.04 JP2.8
N$58  (via drill 0.6)
  Top 0.406: v24.13,77.47 24.13,72.39 29.21,67.31 29.21,58.42 29.54,58.09 OPTO4.16 34.93,57.79 35.56,57.15 R40.2
  Bottom 0.406: v24.13,77.47 JP2.10
N$59
  Top 1.016: Q8.4 86.99,12.06 86.36,12.7 R16.2
N$60  (via drill 0.6)
  Top 0.406: v12.7,25.4 R25.2
  Bottom 0.406: X2.3 12.68,25.38 v12.7,25.4
N$61  (via drill 0.6)
  Top 0.406: v12.7,30.48 R26.2
  Bottom 0.406: X2.4 12.68,30.46 v12.7,30.48
N$62  (via drill 0.6)
  Top 0.406: v12.7,35.56 R27.2
  Bottom 0.406: X2.5 12.68,35.54 v12.7,35.56
N$63  (via drill 0.6)
  Top 0.406: v12.7,40.64 R28.2
  Bottom 0.406: X2.6 12.68,40.62 v12.7,40.64
N$64  (via drill 0.6)
  Top 0.406: v12.7,45.72 R29.2
  Bottom 0.406: X2.7 12.68,45.7 v12.7,45.72
N$65  (via drill 0.6)
  Top 0.406: v12.7,50.8 R30.2
  Bottom 0.406: X2.8 12.68,50.78 v12.7,50.8
N$66  (via drill 0.6)
  Top 0.406: v12.7,55.88 R31.2
  Bottom 0.406: X2.9 12.68,55.86 v12.7,55.88
N$67  (via drill 0.6)
  Top 0.406: v12.7,60.96 R32.2
  Bottom 0.406: X2.10 12.68,60.94 v12.7,60.96
N$68  (via drill 0.6)
  Top 0.406: R33.1 R34.1 R35.1 R36.1 R37.1 R38.1 R39.1 R40.1 40.32,75.25 v38.1,77.47
  Bottom 0.406: v38.1,77.47 38.1,81.28 36.83,82.55 JP2.1
N$69  (via drill 0.6)
  Top 0.406: OPTO3.9 32.38,28.57 v33.02,27.94 | OPTO3.11 32.89,31.11 v33.02,30.99 | OPTO3.13 32.89,33.66 v33.02,33.53 | OPTO3.15 32.89,36.2 v33.02,36.32 | OPTO4.9 32.64,48.9 v33.02,48.51 | OPTO4.11 32.89,51.44 v33.02,51.31 | OPTO4.13 32.89,53.98 v33.02,53.85 | OPTO4.15 32.89,56.52 v33.02,56.64
  Bottom 0.406: JP2.2 34.29,76.2 33.02,74.93 v33.02,56.64 v33.02,53.85 v33.02,51.31 v33.02,48.51 v33.02,36.32 v33.02,33.53 v33.02,30.99 v33.02,27.94
N$71  (via drill 0.9)
  Top 0.61: 71.74,62.85 71.12,62.23 | C2.1 v120.65,67.31
  Top 1.016: OPTO1.8 C3.1 | OPTO2.8 C4.1 | C5.1 71.74,62.85 | OPTO6.8 C6.1 | OPTO7.8 C7.1 | OPTO8.8 C8.1 | C9.1 OPTO9.8 | OPTO10.8 C10.1
  Top 1.422: 81.28,64.77 78.74,62.23 71.12,62.23 OPTO5.8 66.04,62.23 | OPTO1.8 66.04,82.55 66.04,72.39 | 66.04,72.39 66.04,62.23 | 66.04,62.23 66.04,52.07 | 66.04,52.07 66.04,41.91 | 66.04,41.91 66.04,31.75 | 66.04,31.75 66.04,21.59 | 66.04,21.59 66.04,11.43 OPTO10.8 | OPTO2.8 66.04,72.39 | OPTO6.8 66.04,52.07 | OPTO7.8 66.04,41.91 | OPTO8.8 66.04,31.75 | OPTO9.8 66.04,21.59
  Top 1.676: v120.65,67.31 120.65,66.04 119.38,64.77 118.11,64.77
  Top 2.184: 118.11,64.77 81.28,64.77
  Bottom 1.676: IC1.3 120.65,71.12 v120.65,67.31
N$77  (via drill 0.6)
  Top 0.406: R39.2 36.83,54.61 36.2,55.25 OPTO4.14 28.57,55.25 27.94,55.88 27.94,67.31 22.86,72.39 v22.86,74.93
  Bottom 0.406: JP2.9 22.86,82.55 21.59,81.28 21.59,80.01 22.86,78.74 v22.86,74.93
